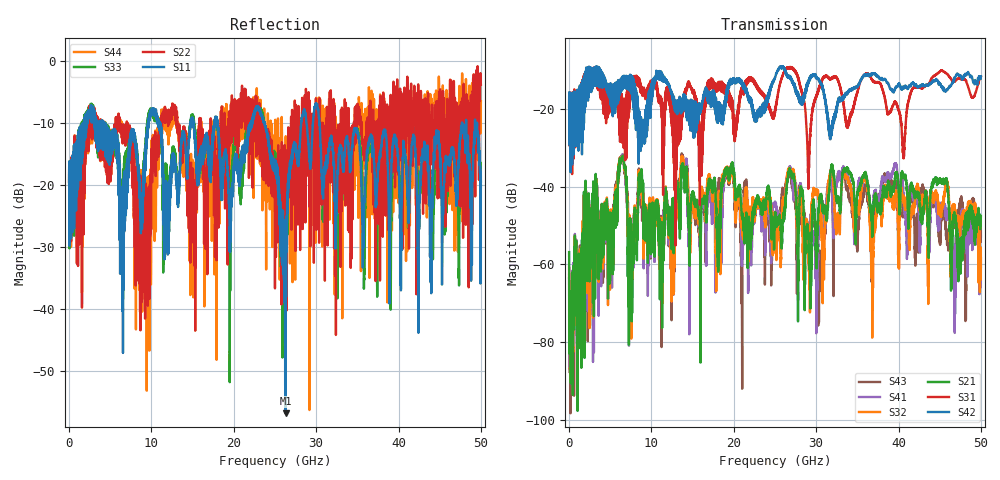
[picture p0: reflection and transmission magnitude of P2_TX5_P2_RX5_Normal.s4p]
!Keysight Technologies,N5225B,MY57041031,A.13.20.10
!Date: Friday, May 31, 2019 11:34:33
!Correction: S11(Full 4 Port(1,2,3,4))
!S12(Full 4 Port(1,2,3,4))
!S13(Full 4 Port(1,2,3,4))
!S14(Full 4 Port(1,2,3,4))
!S21(Full 4 Port(1,2,3,4))
!S22(Full 4 Port(1,2,3,4))
!S23(Full 4 Port(1,2,3,4))
!S24(Full 4 Port(1,2,3,4))
!S31(Full 4 Port(1,2,3,4))
!S32(Full 4 Port(1,2,3,4))
!S33(Full 4 Port(1,2,3,4))
!S34(Full 4 Port(1,2,3,4))
!S41(Full 4 Port(1,2,3,4))
!S42(Full 4 Port(1,2,3,4))
!S43(Full 4 Port(1,2,3,4))
!S44(Full 4 Port(1,2,3,4))
!S4P File: Measurements: <S11,S12,S13,S14>,
!<S21,S22,S23,S24>,
!<S31,S32,S33,S34>,
!<S41,S42,S43,S44>:
# Hz S  dB  R 50.0
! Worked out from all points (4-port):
!   5000 points, 10 MHz to 50 GHz, reference 50 ohm
!   strongest paths, dB at 10 MHz, 12.51 GHz, 25.01 GHz, 37.51 GHz, 50 GHz:
!     S42: -19.5, -16.8, -11.8, -11.5, -11.6
!     S31: -19.4, -17.7, -20.9, -13.1, -11.7
!     S21: -56.8, -48.4, -46.6, -45.7, -47.5
!     S32: -60.8, -49.1, -47.0, -44.7, -58.4
!     S41: -63.6, -49.5, -43.8, -44.4, -60.6
!     S43: -62.5, -51.2, -47.1, -42.6, -52.8
!   lowest |S11| = -56.8 dB at 26.29 GHz (marker M1), VSWR 1.00, Z = 50.1 - j0.0913 ohm
!   |S11| at or under -10 dB: 4.282 GHz to 9.568 GHz (5.286 GHz wide, 76.3 % of centre); 23.74 GHz to 28.18 GHz (4.44 GHz wide, 17.1 % of centre); 30.41 GHz to 47.7 GHz (17.29 GHz wide, 44.3 % of centre)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
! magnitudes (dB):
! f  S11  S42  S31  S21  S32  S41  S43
! 10 MHz  -19.8  -19.5  -19.4  -56.8  -60.8  -63.6  -62.5
! 6.37 GHz  -22.7  -12.6  -18.2  -33.0  -32.8  -32.7  -32.5
! 7.47 GHz  -11.7  -14.2  -12.5  -51.4  -51.9  -52.4  -53.7
! 26.29 GHz  -56.8  -10.7  -9.7  -42.7  -41.0  -41.1  -39.5
! 30.01 GHz  -6.8  -11.8  -16.7  -56.8  -40.8  -77.7  -53.2
! 39.6 GHz  -12.4  -14.7  -18.2  -37.6  -41.3  -34.6  -39.1
! 50 GHz  -19.4  -11.6  -11.7  -47.5  -58.4  -60.6  -52.8
